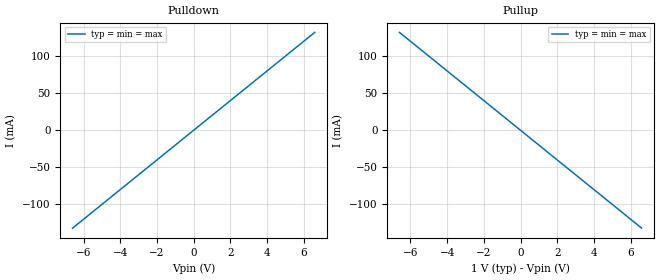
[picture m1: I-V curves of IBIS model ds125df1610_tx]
|Texas Instruments Incorporated
|16 channel retimer with integrated signal conditioning which includes
|an input Continuous-Time Linear Equalizer (CTLE),
|clock and data recovery (CDR)
|and transmit driver on each channel.
| Marketing part#   Voltage Range   Package-type   #pins
| D125DF1610   +2.375 to +2.625   FCBGA   196
[IBIS Ver]   5.1
[File Name]   ds125df1610.ibs
[File Rev]   1.0
[Component]   ds125df1610
[Manufacturer] Texas Instruments
[Disclaimer]
 This product is designed as an aid for customers of Texas Instruments.
 No warranties, either expressed or implied, with respect to this third
 party software (if any) or with respect to its fitness for any
 particular purpose is claimed by Texas Instruments or the author. The
 software (if any) is provided solely on an "as is" basis. The entire
 risk as to its quality and performance is with the customer
[Copyright] (C) Copyright 2017 Texas Instruments Incorporated.
   All rights reserved.
[Package]
R_pkg  0.0   NA   NA
L_pkg  0.0   NA   NA
C_pkg  0.0   NA   NA
[Pin]   signal_name   model_name   R_pin L_pin  C_pin
1p   ds125df1610_tx_p   ds125df1610_tx
1n   ds125df1610_tx_n   ds125df1610_tx
2p   ds125df1610_rx_2p   ds125df1610_rx
2n   ds125df1610_rx_2n   ds125df1610_rx
[Diff_Pin] inv_pin vdiff tdelay_typ tdelay_min tdelay_max
1p   1n   NA   NA   NA   NA
2p   2n   NA   NA   NA   NA
[Model] ds125df1610_rx
Model_type Input
C_comp 0p 0p 0p
Vinh = 0.25
Vinl = -0.25
[Temperature_Range] 25 125 0
[Voltage Range] 1.0 1.0 1.0
[Algorithmic Model]
Executable Windows_cl16.00.40219.01_64 ds125df1610_rx_x64.dll ds125df1610_rx.ami
|Executable Windows_cl16.00.40219.01_32 ds125df1610_rx.dll ds125df1610_rx.ami
|Executable Linux_gcc4.7.2_64 ds125df1610_rx_x64.so ds125DF1610_rx.ami
[End Algorithmic Model]
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| Models and submodels in the file (2): ds125df1610_tx (Output), ds125df1610_rx (Input)
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[Model] ds125df1610_tx
Model_type Output
C_comp 0p 0p 0p
Cref = 0
Vref = 0.5
Rref = 50
Vmeas = 0.5
[Temperature_Range] 25 125 0
[Voltage Range] 1.0 1.0 1.0
[Algorithmic Model]
Executable Windows_cl16.00.40219.01_64 ds125df1610_tx_x64.dll ds125df1610_tx.ami
|Executable Windows_cl16.00.40219.01_32 ds125df1610_tx.dll ds125df1610_tx.ami
|Executable Linux_gcc4.7.2_64 ds125df1610_tx_x64.so ds125df1610_tx.ami
[End Algorithmic Model]
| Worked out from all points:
|   slope of the pulldown table from 0 to 0.15 V, typ, clamps not added: 50 ohm
|   slope of the pullup table from 0 to 0.15 V, typ, clamps not added: 50 ohm
[Pulldown]
-6.6V     -132mA     -132mA     -132mA
0V        0A         0A         0A
6.6V      132mA      132mA      132mA
[Pullup]
-6.6V     132mA      132mA      132mA
0V        0A         0A         0A
6.6V      -132mA     -132mA     -132mA
[GND Clamp]
-6.6V     0A         0A         0A
0V        0A         0A         0A
6.6V      0A         0A         0A
[Power Clamp]
-6.6V     0A         0A         0A
0V        0A         0A         0A
6.6V      0A         0A         0A
[Ramp]
dV/dt_r 0.3/1.5p 0.3/1.5p 0.3/1.5p
dV/dt_f 0.3/1.5p 0.3/1.5p 0.3/1.5p
